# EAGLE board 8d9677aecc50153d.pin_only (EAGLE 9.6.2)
REV: B

Size 50.8 x 22.23 mm. Coordinates in mm from the lower left corner, seen from the top.
Outline: 0.01,0.04 50.8,0 50.8,22.23 0,22.23 0.01,0.04
Copper layers (1*16): Top 0.035mm / dielectric 1.5mm / Bottom 0.035mm
Design rules "adafruit 8-8": minimum track width 6mil, minimum drill 15.5mil, track to track 8mil, track to pad 8mil, pad to pad 8mil, via to via 8mil, smd to smd 8mil, copper to edge 10mil, drill to drill 8mil, minimum pad ring 10mil, minimum via ring 8mil, stop-mask expansion 2mil, vias tented up to drill 20mil, thermal gap 10mil
Net classes: 1 highpower: width 0.305 mm, drill 0.483 mm; 2 lowpower: width 0.254 mm, drill 0.483 mm
Holes 2.8 mm at 47.62,19.74 2.54,2.54

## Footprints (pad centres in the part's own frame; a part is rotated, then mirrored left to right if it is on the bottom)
SOLDERJUMPER_ARROW_NOPASTE = smd 0.762 x 1.524: 1 -1.016,0; 2 1.016,0
0603-NO = smd 1.075 x 1: 1 -0.85,0; 2 0.85,0
0805-NO = smd 1.24 x 1.5: 1 -0.95,0; 2 0.95,0
JST_SH4 = smd 0.6 x 1.55: 1 -1.5,2.006; 2 -0.5,2.006; 3 0.5,2.006; 4 1.5,2.006 | smd 1.2 x 1.8: MT1 -2.8,-1.894; MT2 2.8,-1.894
CHIPLED_0603_NOOUTLINE = smd 0.8 x 0.8: A 0,-0.75; C 0,0.75
SO18W = smd 0.6 x 2.2: 1 -5.095,-4.6; 2 -3.825,-4.6; 3 -2.555,-4.6; 4 -1.285,-4.6; 5 -0.015,-4.6; 6 1.255,-4.6; 7 2.525,-4.6; 8 3.795,-4.6; 9 5.065,-4.6; 10 5.125,4.6; 11 3.855,4.6; 12 2.585,4.6; 13 1.315,4.6; 14 0.045,4.6; 15 -1.225,4.6; 16 -2.495,4.6; 17 -3.795,4.6; 18 -5.095,4.6
SO16 = smd 0.66 x 2.032: 1 -4.445,-3.073; 2 -3.175,-3.073; 3 -1.905,-3.073; 4 -0.635,-3.073; 5 0.635,-3.073; 6 1.905,-3.073; 7 3.175,-3.073; 8 4.445,-3.073; 9 4.445,3.073; 10 3.175,3.073; 11 1.905,3.073; 12 0.635,3.073; 13 -0.635,3.073; 14 -1.905,3.073; 15 -3.175,3.073; 16 -4.445,3.073
SOT23-6 = smd 0.55 x 1.2: 1 -0.95,-1.3; 2 0,-1.3; 3 0.95,-1.3; 4 0.95,1.3; 5 0,1.3; 6 -0.95,1.3
1X05-3.5MM = drill 1 pad 2.184: 1 7,0; 2 3.5,0; 3 0,0; 4 -3.5,0; 5 -7,0
1X16 = drill 1.016 long: 1 -19.05,0; 2 -16.51,0; 3 -13.97,0; 4 -11.43,0; 5 -8.89,0; 6 -6.35,0; 7 -3.81,0; 8 -1.27,0; 9 1.27,0; 10 3.81,0; 11 6.35,0; 12 8.89,0; 13 11.43,0; 14 13.97,0; 15 16.51,0; 16 19.05,0
SOT363 = smd 0.5 x 0.5: 1 -0.75,-0.9; 3 0.75,-0.9; 4 0.75,0.9; 6 -0.75,0.9 | smd 0.4 x 0.5: 2 0,-0.9; 5 0,0.9
RTRIM3314J = smd 1.778 x 1.3: 1 1.492,-1.883; 3 -1.556,-1.927 | smd 2 x 2: 2 0,2
RESPACK_4X0603 = smd 0.45 x 0.9: 1 -1.3,-0.85; 2 -0.4,-0.85; 3 0.4,-0.85; 4 1.3,-0.85; 5 1.3,0.85; 6 0.4,0.85; 7 -0.4,0.85; 8 -1.3,0.85
SOLDERJUMPER_CLOSEDWIRE = smd 1.168 x 1.6: 1 -0.762,0; 2 0.762,0 | smd 0.635 x 0.203: WIRE 0,0
TESTPOINT_ROUND_1.5MM = smd 1.5 x 1.5: P$1 0,0
FIDUCIAL_1MM = smd 1 x 1: 1 0,0

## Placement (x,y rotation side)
A0  [SOLDERJUMPER_ARROW_NOPASTE]  17.27,3.05 0 top
A1  [SOLDERJUMPER_ARROW_NOPASTE]  13.46,3.05 0 top
A2  [SOLDERJUMPER_ARROW_NOPASTE]  9.53,3.05 0 top
C1  0.1uF  [0603-NO]  30.23,9.4 90 top
C2  0.1uF  [0603-NO]  5.59,16.13 270 top
C4  10uF  [0805-NO]  33.53,12.06 180 top
C5  10uF  [0805-NO]  42.04,12.45 180 top
C6  1uF  [0805-NO]  30.61,14.48 270 top
CONN3  STEMMA_I2C_QT  [JST_SH4]  22.73,3.43 0 top
CONN4  STEMMA_I2C_QT  [JST_SH4]  47.37,14.22 90 top
D1  GREEN  [CHIPLED_0603_NOOUTLINE]  49.4,9.27 0 top
IC1  MCP23008/SO  [SO18W]  12.59,10.41 0 top
IC2  74HC595D  [SO16]  24.13,11.81 180 top
IC3  AP3602/RT9361  [SOT23-6]  33.66,14.48 90 top
J1  1X5  [1X05-3.5MM]  40.89,3.81 0 top
JP1  [1X16]  23.11,19.74 180 top
PLABEL0  [PLABEL0]  45.21,7.49 90 top
PLABEL1  [PLABEL1]  48.39,7.37 90 top
PLABEL2  [PLABEL2]  37.97,7.62 90 top
PLABEL3  [PLABEL3]  41.4,7.62 90 top
PLABEL4  [PLABEL4]  34.29,7.75 90 top
PLABEL5  [PLABEL5]  8.38,0.64 0 top
PLABEL6  [PLABEL6]  12.45,0.76 0 top
PLABEL7  [PLABEL7]  16.51,0.76 0 top
PLABEL8  [PLABEL8]  29.02,2.35 0 top
PLABEL9  [PLABEL9]  1.27,6.73 90 top
PLABEL10  [PLABEL10]  6.99,16.51 0 top
PLABEL11  [PLABEL11]  29.02,1.08 0 top
PLABEL12  [PLABEL12]  46.48,6.6 0 bottom
Q1  BSS138  [SOT363]  3.24,16.19 0 top
Q2  BSS138  [SOT363]  42.04,14.86 270 top
R1  10K  [0603-NO]  46.1,9.27 270 top
R2  3314J-1-104E  [RTRIM3314J]  3.81,7.49 0 top
R3  4.7K Pack  [RESPACK_4X0603]  37.97,14.61 270 top
R6  10K  [0603-NO]  28.96,3.68 180 top
R8  4.7K Pack  [RESPACK_4X0603]  4.57,12.57 270 top
SJ1  [SOLDERJUMPER_CLOSEDWIRE]  42.67,9.4 90 top
SPIEN  [SOLDERJUMPER_ARROW_NOPASTE]  28.83,5.59 0 top
TP1  [TESTPOINT_ROUND_1.5MM]  9.27,3.05 0 bottom
TP2  [TESTPOINT_ROUND_1.5MM]  13.21,3.05 0 bottom
TP3  [TESTPOINT_ROUND_1.5MM]  17.27,3.05 0 bottom
TP4  [TESTPOINT_ROUND_1.5MM]  28.83,5.33 0 bottom
U$1  FIDUCIAL  [FIDUCIAL_1MM]  1.52,20.83 0 top
U$2  FIDUCIAL  [FIDUCIAL_1MM]  46.1,5.84 0 top
U$4  [ADAFRUIT_3.5MM]  3.94,0.38 0 top
U$7  [PCBFEAT-REV-040]  30.73,17.27 0 top
U$11  [STEMMAQT]  47.88,9.27 90 bottom
U$12  [STEMMAQT]  27.69,0.25 0 bottom
U$23  [ADAFRUIT_TEXT_20MM]  20.19,10.29 0 bottom

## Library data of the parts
A0 A1 A2 SPIEN = microbuilder; BOM: EXCLUDE
C1 C2 C4-C6 R1 R3 R6 R8 SJ1 TP1-TP4 U$4 U$7 U$23 = microbuilder
CONN3 CONN4 = adafruit_electromech; LCSC: C2845363
D1 IC3 = microbuilder; ROT: 270
IC1 J1 U$1 U$2 = adafruit
IC2 = 74xx-us
JP1 = pinhead
PLABEL0 PLABEL1-PLABEL12 = pinguin
Q1 Q2 = microbuilder; JLC_ROTATION: 270
R2 = adafruit_electromech; SPICEMODEL: X; SPICEPREFIXL: POT
U$11 U$12 = silks

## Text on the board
Pinguin_tBackup: I2C / SPI LCD backpack | Contrast | LAT | DAT | CLK | 3-5V | GND | SPI | A2 | A1 | A0 | Enable
Pinguin_bBackup: I2C or SPI / Character LCD Backpack / Vin/Vlogic: 3~5V DC

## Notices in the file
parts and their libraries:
microbuilder: This work is placed in the public domain, and may be freely used for commercial and non-commercial work with the following conditions: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
